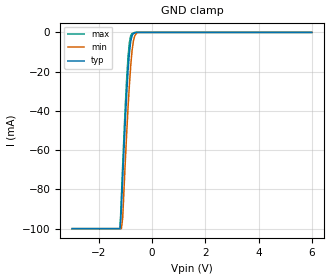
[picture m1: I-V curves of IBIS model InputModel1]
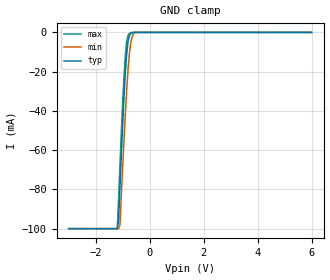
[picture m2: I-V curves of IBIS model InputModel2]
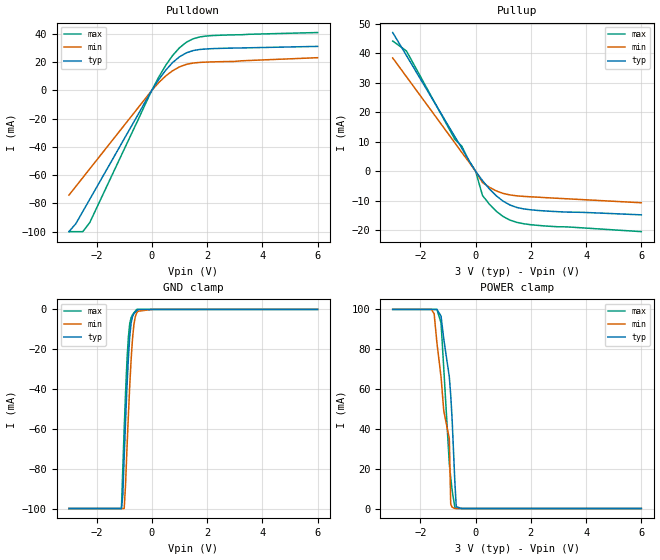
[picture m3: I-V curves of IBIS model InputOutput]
[IBIS Ver]   2.1
[File name]   pa016scl.ibs   | pa= PSOP, f016sc-l= abbr chip name,
|   | l = 2.7 to 3.3 Vcc
[File Rev]   2.00
[Date]   18-April-1996
[Source]   File generated from lab measurements at Intel Corporation
[Notes]   Rev 2.00 All data was replaced by actual measurements
   performed in a lab.
[Disclaimer] INTEL DEVELOPER'S SOFTWARE LICENSE AGREEMENT
| BY USING THIS SOFTWARE, YOU ARE AGREEING TO BE BOUND
| BY THE TERMS OF THIS AGREEMENT.  DO NOT USE THE SOFTWARE
| UNTIL YOU HAVE CAREFULLY READ AND AGREED TO THE FOLLOWING
| TERMS AND CONDITIONS.  IF YOU DO NOT AGREE TO THE TERMS
| OF THIS AGREEMENT, PROMPTLY RETURN THE SOFTWARE PACKAGE
| AND ANY ACCOMPANYING ITEMS.
| IF YOU USE THIS SOFTWARE, YOU WILL BE BOUND BY THE TERMS
| OF THIS AGREEMENT
| LICENSE: Intel Corporation ("Intel") grants you the non-exclusive right
| to use the enclosed software program ("Software").  You will not use,
| copy, modify, rent, sell or transfer the Software or any portion
| thereof, except as provided in this Agreement.
| System OEM Developers may:
| 1.   Copy the Software for support, backup or archival purposes;
| 2.   Install, use, or distribute Intel owned Software in object code
|   only;
| 3.   Modify and/or use Software source code that Intel directly makes
|   available to you as an OEM Developer;
| 4.   Install, use, modify, distribute, and/or make or have made
|   derivatives ("Derivatives") of Intel owned Software under the
|   terms and conditions in this Agreement, ONLY if you are a System
|   OEM Developer and NOT an end-user.
| RESTRICTIONS:
| YOU WILL NOT:
| 1.   Copy the Software, in whole or in part, except as provided for
|   in this Agreement;
| 2.   Decompile or reverse engineer any Software provided in object
|   code format;
| 3.   Distribute any Software or Derivative code to any end-users,
|   unless approved by Intel in a prior writing.
| TRANSFER: You may transfer the Software to another OEM
| Developer if the receiving party agrees to the terms of this
| Agreement at the sole risk of any receiving party.
| OWNERSHIP AND COPYRIGHT OF SOFTWARE:
| Title to the Software and all copies thereof remain with Intel
| or its vendors.  The Software is copyrighted and is protected by
| United States and international copyright laws.  You will not
| remove the copyright notice from the Software.  You agree to
| prevent any unauthorized copying of the Software.
| DERIVATIVE WORK: OEM Developers that make or have made
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[Copyright]   Copyright 1996, Intel Corporation, All Rights Reserved
[Component]   PA28F016SC-L   | 44-lead PSOP package, 28F016SC-L
[Manufacturer]  Intel   | Flash File (tm)
|   | operating in 2.7 to 3.3 V Vcc range
[Package]
|The following values apply for the leadframe.
|Variable   typ   min   max
R_pkg   145m   144m   147m
L_pkg   5.25nH   2.00nH   8.50nH
C_pkg   1.09pF   0.68pF   1.50pF
|*****************************Pin Definitions**********************************
[Pin]   signal_name   model_name   R_pin   L_pin   C_pin
  1   VPP   POWER
  2   RP#   InputModel1
  3   A11   InputModel1
  4   A10   InputModel1
  5   A09   InputModel1
  6   A08   InputModel1
  7   A07   InputModel1
  8   A06   InputModel1
  9   A05   InputModel1
 10   A04   InputModel1
 11   NC   InputModel2
 12   NC   InputModel2
 13   A03   InputModel1
 14   A02   InputModel1
 15   A01   InputModel1
 16   A00   InputModel1
 17   DQ0   InputOutput
 18   DQ1   InputOutput
 19   DQ2   InputOutput
 20   DQ3   InputOutput
 21   GND   GND
 22   GND   GND
 23   VCC   POWER
 24   DQ4   InputOutput
 25   DQ5   InputOutput
 26   DQ6   InputOutput
 27   DQ7   InputOutput
 28   RY/BY#   RYBYOutput
 29   OE#   InputModel2
 30   WE#   InputModel2
 31   NC   InputModel2
 32   NC   InputModel2
 33   NC   InputModel2
 34   A20   InputModel1
 35   A19   InputModel1
 36   A18   InputModel1
 37   A17   InputModel1
 38   A16   InputModel1
 39   A15   InputModel1
 40   A14   InputModel1
 41   A13   InputModel1
 42   A12   InputModel1
 43   CE#   InputModel1
 44   VCC   POWER
| Models and submodels in the file (4): InputModel1 (Input), InputModel2 (Input), InputOutput (I/O), RYBYOutput (Output)
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|**************************Input Model 1***************************************
[Model]   InputModel1
Model_type   Input
|   For A[0:20], CE# & RP#
Vinl = 0.8V
Vinh = 2.0V
| Variable   typ   min   max
C_comp   5.61p   NA   7.6p
[Voltage Range]   3.0V   2.7V   3.3V
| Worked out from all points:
|   GND clamp passes 1 mA (typ) near -0.72 V on its own axis
[GND_clamp]
|Voltage I(typ)   I(min)   I(max)
-3V       -100mA     -100mA     -100mA
-1.2V     -100mA     -100mA     -100mA
-1.15V    -89.78mA   -100mA     -83.95mA
-1.1V     -73.97mA   -94.36mA   -67.26mA
-950mV    -31.34mA   -51.06mA   -23.34mA
-900mV    -19.72mA   -38.17mA   -12.45mA
-850mV    -10.75mA   -26.88mA   -5.276mA
-800mV    -4.602mA   -16.94mA   -1.691mA
-750mV    -1.638mA   -9.411mA   -584.3uA
-650mV    -256.1uA   -1.87mA    0A
-550mV    0A         0A         0A
6V        0A         0A         0A
[POWER_clamp]
| Input buffer circuits of this product do not intrinsically
| require a [POWER_clamp] definition.  This zero current
| [POWER_clamp] is provided for compatibility with some ibis
| parsers.
|Voltage  I(typ)   I(min)   I(max)
-3V       0A         0A         0A
0V        0A         0A         0A
3V        0A         0A         0A
6V        0A         0A         0A
|**********************Input Model 2************************************
[Model]   InputModel2
Model_type   Input
|   For OE#, WE#, NC Pins
Vinl = 0.8V
Vinh = 2.0V
| Variable   typ   min   max
C_comp   5.61p   NA   7.6p
[Voltage Range]   3.0V   2.7V   3.3V
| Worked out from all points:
|   GND clamp passes 1 mA (typ) near -0.72 V on its own axis
[GND_clamp]
|Voltage I(typ)   I(min)   I(max)
-3V       -100mA     -100mA     -100mA
-1.2V     -100mA     -100mA     -100mA
-1.15V    -95.58mA   -100mA     -85.14mA
-1.1V     -78.87mA   -98.11mA   -67.9mA
-950mV    -32.87mA   -54.74mA   -22.48mA
-900mV    -20.42mA   -41.3mA    -11.63mA
-850mV    -10.96mA   -29.41mA   -4.661mA
-800mV    -4.607mA   -18.84mA   -1.461mA
-750mV    -1.626mA   -10.73mA   -518.6uA
-650mV    -251.5uA   -2.311mA   0A
-550mV    0A         0A         0A
6V        0A         0A         0A
[POWER_clamp]
| Input buffer circuits of this product do not intrinsically
| require a [POWER_clamp] definition.  This zero current
| [POWER_clamp] is provided for compatibility with some ibis
| parsers.
|Voltage  I(typ)   I(min)   I(max)
-3V       0A         0A         0A
0V        0A         0A         0A
3V        0A         0A         0A
6V        0A         0A         0A
|**************************Input Output Model*********************************
[Model]   InputOutput
Model_type   I/O
|   for DQ[0:7]
Vinl = 0.8V
Vinh = 2.0V
| Variable   typ   min   max
C_comp   9.61p   NA   11.6p
[Voltage Range]   3.0V   2.7V   3.3V
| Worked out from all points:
|   slope of the pulldown table from 0 to 0.45 V, typ, clamps not added: 35 ohm
|   slope of the pullup table from 0 to 0.45 V, typ, clamps not added: 82.7 ohm
|   GND clamp passes 1 mA (typ) near -0.58 V on its own axis
|   POWER clamp passes 1 mA (typ) near -0.70 V on its own axis
[Pulldown]
| [Pullup] and [Pulldown] IV curves include only the current through
| the channels of output driver transistors when outputs are enabled
| with OE# = VIL.  Although the output driver transistors have np and
| pn diodes inherently created by CMOS IC fabrication between the
| drain and bulk of n-channel and p-channel CMOS transistors,
| the current through these junction diodes is not included in
| [Pullup] or [Pulldown].  Instead that drain/bulk diode current is
| included in the [POWER_clamp] or [GND_clamp] sections, which are
| not dependent on the state of OE# or output data value.
|Voltage  I(typ)   I(min)   I(max)
-3V       -100mA     -74.16mA   -100mA
-2.75V    -94.37mA   -67.99mA   -100mA
-2.5V     -85.79mA   -61.81mA   -100mA
-2.25V    -77.22mA   -55.64mA   -93.7mA
0V        0A         0A         0A
250mV     7.606mA    5.483mA    9.324mA
750mV     19.59mA    13.84mA    24.6mA
1V        23.73mA    16.61mA    30.1mA
1.25V     26.53mA    18.38mA    34.03mA
1.5V      28.17mA    19.33mA    36.52mA
2V        29.33mA    20.01mA    38.48mA
6V        31.1mA     23.1mA     40.9mA
[GND_clamp]
| [POWER_clamp] and [GND_clamp] IV curves describe ESD protection
| circuits PLUS some np and pn diodes which exist between the
| drain and bulk of n-channel and p-channel CMOS transistors.
| These drain/bulk diodes are inherent in CMOS IC fabrication,
| and are visible on the node of the I/O pin at all times.
| Even the drain/bulk diodes of output driver [Pullup] and [Powerdown]
| transistors are included in [POWER_clamp] or [GND_clamp], because
| these diodes contribute to I/O pin current even when the
| chip outputs are tristated by OE# = VIH.
| For example, when V forced on the I/O pin is large, we are
| forward biasing the pn diode at the drain/bulk interface in the
| p-channel pullup transistor.  Similarly, when V forced on the
| I/O pin is sufficiently negative with respect to the substrate
| ground, we are forward biasing the np diode at the drain/bulk
| interface in the n-channel pulldown transistor.  The effects
| of these diodes are included in [POWER_clamp] or [GND_clamp].
|Voltage  I(typ)   I(min)   I(max)
-3V       -100mA     -100mA     -100mA
-1.1V     -100mA     -100mA     -100mA
-1.05V    -93.3mA    -100mA     -79.79mA
-1V       -73.94mA   -100mA     -59.86mA
-950mV    -55.77mA   -87.63mA   -41.64mA
-900mV    -38.86mA   -69.89mA   -25.76mA
-850mV    -24.81mA   -53.69mA   -14.14mA
-800mV    -13.64mA   -38.37mA   -7.148mA
-700mV    -3.618mA   -14.83mA   -2.683mA
-650mV    -2.146mA   -7.792mA   -1.704mA
-550mV    -701.9uA   -1.814mA   0A
6V        0A         0A         0A
[Pullup]
| (Voltages for [Pullup] and [POWER_clamp] are specified with
| negative respect to Vcc.  Reference the IBIS documentation
| for more information regarding Vtable = Vcc - Voutput.
| This method keeps -Vds constant for the values in all three
| columns across a line of the table.
| [Pullup] and [Pulldown] IV curves include only the current through
| the channels of output driver transistors when outputs are enabled
| with OE# = VIL.  Although the output driver transistors have np and
| pn diodes inherently created by CMOS IC fabrication between the
| drain and bulk of n-channel and p-channel CMOS transistors,
| the current through these junction diodes is not included in
| [Pullup] or [Pulldown].  Instead that drain/bulk diode current is
| included in the [POWER_clamp] or [GND_clamp] sections, which are
| not dependent on the state of OE# or output data value.
|Voltage  I(typ)   I(min)   I(max)
-3V       47.05mA    38.43mA    44.17mA
-2.5V     39.2mA     32.03mA    40.75mA
-750mV    11.73mA    9.63mA     10.83mA
-500mV    7.839mA    6.381mA    8.528mA
-250mV    3.757mA    3.273mA    3.705mA
0V        0A         0A         0A
250mV     -3.188mA   -3.828mA   -8.223mA
750mV     -8.346mA   -6.683mA   -13.58mA
1V        -10.18mA   -7.536mA   -15.39mA
1.5V      -12.32mA   -8.357mA   -17.37mA
2V        -13.09mA   -8.686mA   -18.15mA
6V        -14.8mA    -10.7mA    -20.5mA
[POWER_clamp]
| (Voltages for [Pullup] and [POWER_clamp] are specified with
| negative respect to Vcc.  Reference the IBIS documentation
| for more information regarding Vtable = Vcc - Voutput.
| This method keeps -Vds constant for the values in all three
| columns across a line of the table.
| [POWER_clamp] and [GND_clamp] IV curves describe ESD protection
| circuits PLUS some np and pn diodes which exist between the
| drain and bulk of n-channel and p-channel CMOS transistors.
| These drain/bulk diodes are inherent in CMOS IC fabrication,
| and are visible on the node of the I/O pin at all times.
| Even the drain/bulk diodes of output driver [Pullup] and [Powerdown]
| transistors are included in [POWER_clamp] or [GND_clamp], because
| these diodes contribute to I/O pin current even when the
| chip outputs are tristated by OE# = VIH.
| For example, when V forced on the I/O pin is large, we are
| forward biasing the pn diode at the drain/bulk interface in the
| p-channel pullup transistor.  Similarly, when V forced on the
| I/O pin is sufficiently negative with respect to the substrate
| ground, we are forward biasing the np diode at the drain/bulk
| interface in the n-channel pulldown transistor.  The effects
| of these diodes are included in [POWER_clamp] or [GND_clamp].
|Voltage  I(typ)   I(min)   I(max)
-3V       100mA      100mA      100mA
-1.6V     100mA      100mA      100mA
-1.5V     100mA      97.85mA    100mA
-1.4V     100mA      83.31mA    100mA
-1.25V    96.63mA    66mA       93.28mA
-1.15V    85mA       48.89mA    70mA
-950mV    66mA       35mA       22.25mA
-900mV    57mA       2.263mA    15.61mA
-850mV    45mA       668.3uA    9.3mA
-750mV    13.3mA     0A         593.8uA
-700mV    879uA      0A         0A
6V        0A         0A         0A
[Ramp]
| The DQ Ramp information is not provided at this time for the
| device but will be available in the future.  The table below
| is for the compatibility with some IBIS parsers.
| Variable   typ   min   max
 dV/dt_r   0V/0ns   0V/0ns   0V/0ns
 dV/dt_f   0V/0ns   0V/0ns   0V/0ns
